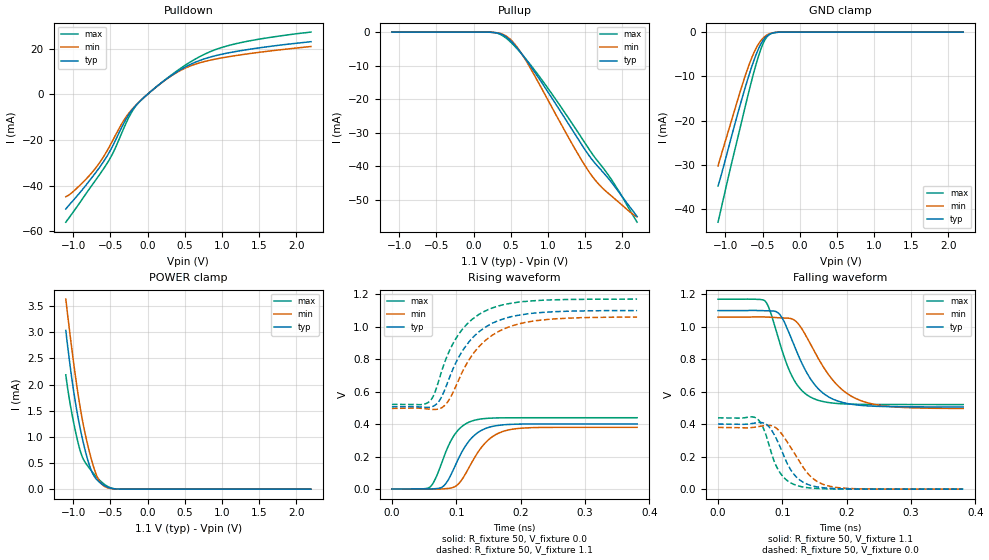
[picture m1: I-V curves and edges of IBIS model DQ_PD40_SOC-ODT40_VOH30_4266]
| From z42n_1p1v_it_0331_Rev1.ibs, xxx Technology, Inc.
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| DQ_PD40_SOC-ODT40_VOH30_4266
| (40 Ohm Pulldown, 40 Ohm System ODT Setting, VOH=VDDQ/3.0, 3200-4266Mbps)
[Model]   DQ_PD40_SOC-ODT40_VOH30_4266
Model_type   I/O
Vinl = 123.333mV
Vinh = 243.333mV
Vmeas = 183.333mV
Vref = 0.0mV
Cref = 0.0pF
Rref = 40.000Ohm
|   typ   min   max
|C_comp   0.834pF   0.784pF   0.884pF
C_comp_pullup   0.4170pF   0.3920pF   0.4420pF
C_comp_pulldown   0.4170pF   0.3920pF   0.4420pF
| Note: C_comp changes when the ODT circuit is enabled.
[Model Spec]
| Input threshold voltage corners
Vinl   0.1233V   0.1167V   0.1350V
Vinh   0.2433V   0.2367V   0.2550V
| Measurement voltage corners
Vmeas   0.1833V   0.1767V   0.1950V
| Timing spec test load voltage corners
Vref   0.0000V   0.0000V   0.0000V
| Dynamic Overshoot Parameters from LPDDR4 Specification
D_overshoot_ampl_h   0.30   NA   NA
D_overshoot_ampl_l   0.30   NA   NA
D_overshoot_area_h   0.1n   NA   NA
D_overshoot_area_l   0.1n   NA   NA
[Voltage Range]   1.1000V   1.0600V   1.1700V
[Pullup Reference]   1.1000V   1.0600V   1.1700V
| Junction Temperature (Ambient temp is 35C typ 95C min -40C max)
[Temperature Range]   50.0   110.0   -40.0
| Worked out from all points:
|   slope of the pulldown table from 0 to 0.165 V, typ, clamps not added: 36.9 ohm
|   slope of the pullup table from 0 to 0.165 V, typ, clamps not added: 13.1 kohm
|   GND clamp passes 1 mA (typ) near -0.45 V on its own axis
|   POWER clamp passes 1 mA (typ) near -0.88 V on its own axis
|   rising waveform, R_fixture 50, V_fixture 0.0: 20-80 % time 34.6ps typ, 38.5ps min, 30.1ps max; typ from 0.001 V to 0.401 V
|   falling waveform, R_fixture 50, V_fixture 1.1: 20-80 % time 45.8ps typ, 57.5ps min, 35.9ps max; typ from 1.1 V to 0.507 V
|   rising waveform, R_fixture 50, V_fixture 1.1: 20-80 % time 55.8ps typ, 59.1ps min, 51.8ps max; typ from 0.507 V to 1.1 V
|   falling waveform, R_fixture 50, V_fixture 0.0: 20-80 % time 31.1ps typ, 39.2ps min, 25.8ps max; typ from 0.401 V to 0.001 V
[Pulldown]
|   Voltage   I(typ)   I(min)   I(max)
-1.1V     -50.2mA    -44.82mA   -55.96mA
-885.5mV  -42.07mA   -39.05mA   -46.22mA
-684.2mV  -33.7mA    -31.69mA   -36.93mA
-479.6mV  -23.26mA   -20.91mA   -26.61mA
-314.6mV  -12.44mA   -11.23mA   -14.52mA
-176mV    -5.609mA   -5.442mA   -5.939mA
-44mV     -1.309mA   -1.3mA     -1.284mA
272.8mV   7.088mA    6.98mA     7.23mA
573.1mV   12.96mA    12.33mA    14.03mA
1.009V    17.56mA    15.95mA    20.54mA
1.434V    19.96mA    18.04mA    23.71mA
2.2V      22.98mA    20.89mA    27.18mA
[GND Clamp]
|   Voltage   I(typ)   I(min)   I(max)
-1.1V     -34.74mA   -30.21mA   -42.91mA
-1.05V    -31.86mA   -27.33mA   -39.27mA
-941.6mV  -25.02mA   -21.26mA   -31.32mA
-799.7mV  -16.31mA   -13.32mA   -21.42mA
-667.7mV  -8.907mA   -6.722mA   -12.29mA
-595.1mV  -5.399mA   -3.899mA   -7.689mA
-522.5mV  -2.664mA   -1.902mA   -3.812mA
-473mV    -1.421mA   -1.031mA   -1.888mA
-416.9mV  -604.9uA   -440.1uA   -666.1uA
-354.2mV  -179.2uA   -134.5uA   -160uA
-248.6mV  -12.37uA   -10.94uA   -7.168uA
2.2V      0A         0A         0A
[Pullup]
|   Voltage   I(typ)   I(min)   I(max)
-1.1V     6.275uA    9.671uA    2.829uA
226.6mV   -42.05uA   -43.01uA   -42.87uA
342.1mV   -380.5uA   -313.4uA   -524.7uA
437.8mV   -1.437mA   -1.177mA   -1.807mA
553.3mV   -3.879mA   -3.574mA   -4.208mA
695.2mV   -7.909mA   -8.165mA   -7.815mA
955.9mV   -16.38mA   -18.46mA   -15.4mA
1.322V    -28.99mA   -33.23mA   -27.17mA
1.586V    -37.82mA   -42.74mA   -36.02mA
1.695V    -40.67mA   -45.67mA   -39.19mA
1.867V    -45.16mA   -49.15mA   -44.41mA
2.2V      -55.05mA   -55.17mA   -56.74mA
[POWER Clamp]
|   Voltage   I(typ)   I(min)   I(max)
-1.1V     3.033mA    3.633mA    2.184mA
-1.041V   2.345mA    2.929mA    1.625mA
-977.9mV  1.723mA    2.241mA    1.16mA
-908.6mV  1.177mA    1.582mA    747uA
-852.5mV  818.3uA    1.148mA    543.5uA
-776.6mV  434.1uA    683.3uA    390.2uA
-713.9mV  239.3uA    373uA      278.6uA
-657.8mV  146.8uA    178.8uA    190.7uA
-595.1mV  80.74uA    68.29uA    109.3uA
-482.9mV  15.72uA    9.483uA    19.49uA
-364.1mV  1.116uA    820nA      867nA
2.2V      0A         0A         0A
[Ramp]
|   typ   min   max
| 20% - 80%
dV/dt_r   240.33m/34.56p   227.87m/38.49p   263.36m/30.08p
dV/dt_f   356.01m/45.76p   337.60m/57.53p   389.19m/35.90p
| 25% - 75%
|dV/dt_r   200.27m/27.53p   189.89m/30.67p   219.46m/23.85p
|dV/dt_f   296.67m/36.50p   281.33m/45.92p   324.32m/28.58p
R_load = 50
[Rising Waveform]
R_fixture = 50
V_fixture = 0.0
|   Time   V(typ)   V(min)   V(max)
0s        555.3uV    475.8uV    405.9uV
58ps      265.4uV    42.33uV    9.634mV
67ps      2.281mV    -539.9uV   58.87mV
78ps      12.17mV    763.2uV    168.8mV
87ps      52.88mV    3.665mV    259.5mV
100ps     158.9mV    20.13mV    349.2mV
127ps     327mV      184mV      422.4mV
152ps     381.8mV    310.2mV    436.5mV
184ps     398.3mV    366.5mV    439.1mV
381ps     401.1mV    380.3mV    439.3mV
[Falling Waveform]
R_fixture   = 50
V_fixture   = 1.1
V_fixture_min = 1.06
V_fixture_max = 1.17
|   Time   V(typ)   V(min)   V(max)
0s        1.1V       1.06V      1.17V
74ps      1.099V     1.06V      1.155V
96ps      1.076V     1.056V     899.7mV
115ps     917.3mV    1.048V     695.5mV
129ps     786.7mV    995.6mV    612.8mV
149ps     649.8mV    853.7mV    557.3mV
183ps     547.6mV    650.8mV    528.7mV
220ps     517mV      548.4mV    522.7mV
274ps     508.1mV    506.7mV    521.5mV
381ps     506.7mV    497.3mV    521.4mV
[Rising Waveform]
R_fixture   = 50
V_fixture   = 1.1
V_fixture_min = 1.06
V_fixture_max = 1.17
|   Time   V(typ)   V(min)   V(max)
0s        506.5mV    496.8mV    521.3mV
57ps      503.2mV    492.5mV    534.9mV
66ps      513.8mV    490mV      587.2mV
79ps      582.3mV    505.1mV    746.8mV
93ps      722mV      579.4mV    881.6mV
111ps     859.4mV    733.7mV    990.9mV
129ps     945.9mV    847.5mV    1.058V
150ps     1.008V     930.4mV    1.106V
222ps     1.084V     1.036V     1.16V
381ps     1.099V     1.059V     1.17V
[Falling Waveform]
R_fixture = 50
V_fixture = 0.0
|   Time   V(typ)   V(min)   V(max)
0s        401.2mV    380.4mV    439.4mV
57ps      407.8mV    381.8mV    442.6mV
66ps      411.1mV    388mV      409.9mV
75ps      399.5mV    393.6mV    328.5mV
95ps      274.2mV    359.7mV    109.8mV
110ps     139.5mV    275.8mV    46.36mV
124ps     66.78mV    187.5mV    21.27mV
147ps     20.1mV     67.74mV    6.235mV
177ps     4.831mV    15.51mV    1.586mV
381ps     605.8uV    554uV      424.5uV
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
